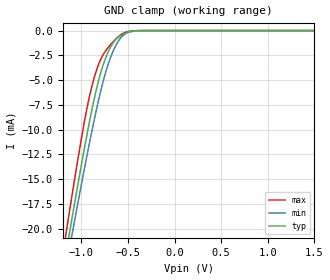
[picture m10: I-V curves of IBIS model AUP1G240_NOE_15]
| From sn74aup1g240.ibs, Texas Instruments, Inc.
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[Model]   AUP1G240_NOE_15
Model_type  Input
Vinl=0.56
Vinh=0.91
| variable   typ   min   max
C_comp   1.68pF   1.45pF   1.91pF
[Temperature Range]   40   100   -40
| Ambient temperature   25   85   -40
[Voltage range]   1.5   1.4   1.6
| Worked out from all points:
|   GND clamp passes 1 mA (typ) near -0.64 V on its own axis
[GND Clamp]
| AUP1G240_NOE_15
|   Voltage   I(typ)   I(min)   I(max)
-3.6V     -171.6mA   -163.5mA   -181.1mA
-1.16V    -22.22mA   -23.69mA   -20.18mA
-1.135V   -20.83mA   -22.39mA   -18.68mA
-1.11V    -19.45mA   -21.09mA   -17.19mA
-1.09V    -18.36mA   -20.06mA   -16.01mA
-955mV    -11.25mA   -13.33mA   -8.55mA
-850mV    -6.372mA   -8.471mA   -4.359mA
-775mV    -3.711mA   -5.429mA   -2.571mA
-705mV    -1.995mA   -3.175mA   -1.611mA
-550mV    -358.9uA   -463.8uA   -270.8uA
-330mV    -2.909uA   -4.637uA   -452.5nA
1.5V      74.87pA    434.2pA    15.81pA
